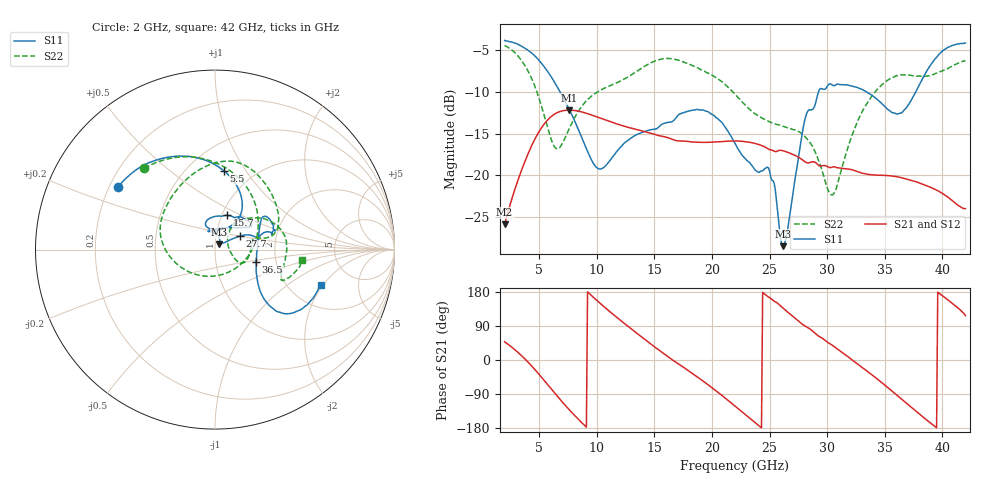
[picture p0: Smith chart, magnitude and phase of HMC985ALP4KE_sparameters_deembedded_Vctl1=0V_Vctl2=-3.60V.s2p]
!s2p File: Measurements: S11, S21, S12, S22
# GHz S dB R 50.0
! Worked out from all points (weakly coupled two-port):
!   401 points, 2 GHz to 42 GHz, reference 50 ohm
!   highest |S21| = -12.18 dB at 7.6 GHz (marker M1); lowest = -25.8 dB at 2 GHz (marker M2)
!   lowest |S11| = -28.5 dB at 26.2 GHz (marker M3), VSWR 1.08, Z = 52.3 + j3.11 ohm
!   |S11| at or under -10 dB: 6.815 GHz to 29.25 GHz (22.44 GHz wide, 124 % of centre); 33.42 GHz to 37.69 GHz (4.274 GHz wide, 12 % of centre)
!   |S22| runs from -22.3 to -4.4 dB; largest |S21 - S12| = 0.00033
!   S11 on the Smith chart (normalised r, x): 2 GHz: 0.24, +0.28; 5.5 GHz: 0.74, +0.80; 15.7 GHz: 1.06, +0.42; 27.7 GHz: 1.30, +0.20; 36.5 GHz: 1.57, -0.23; 42 GHz: 2.94, -1.90
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2  -3.84 146.9  -25.85 48.2  -25.85 48.1  -4.43 131.1
3.6  -4.63 120.0  -18.91 7.6  -18.91 7.6  -6.50 86.4
5.5  -7.10 83.4  -13.73 -56.3  -13.74 -56.3  -13.14 6.6
6.5  -9.23 66.2  -12.52 -92.8  -12.52 -92.8  -16.79 -67.9
7.6  -12.07 54.3  -12.18 -130.9  -12.19 -130.9  -14.43 -139.0
8.7  -15.47 54.6  -12.40 -165.5  -12.40 -165.5  -11.72 -173.2
10.3  -19.24 87.8  -13.13 149.3  -13.12 149.3  -9.80 160.8
12.6  -15.91 109.0  -14.20 91.5  -14.19 91.5  -8.29 127.3
15.4  -14.18 75.6  -15.25 26.3  -15.25 26.2  -6.14 85.0
15.7  -13.85 70.3  -15.31 19.6  -15.32 19.5  -6.04 81.3
19.4  -12.27 33.2  -16.04 -59.4  -16.04 -59.4  -7.57 35.0
22  -16.16 51.4  -15.87 -121.6  -15.88 -121.6  -10.28 12.9
24.9  -19.08 104.5  -16.85 166.4  -16.84 166.4  -13.51 12.0
26.2  -28.47 51.9  -17.05 136.2  -17.06 136.2  -14.13 -4.1
27.7  -16.15 28.7  -17.98 98.0  -17.98 97.9  -14.90 -22.9
28.7  -12.12 12.7  -18.37 77.3  -18.36 77.3  -16.45 -27.8
30.5  -9.22 18.3  -18.98 37.7  -18.99 37.7  -22.31 19.1
32.9  -9.63 33.9  -19.67 -16.7  -19.67 -16.7  -12.75 46.8
35.4  -12.22 11.7  -20.04 -76.1  -20.03 -76.1  -8.48 19.0
36.5  -12.48 -16.6  -20.29 -104.2  -20.29 -104.2  -7.96 6.0
39.5  -5.86 -43.7  -21.76 -178.6  -21.75 -178.7  -7.75 -24.2
42  -4.15 -18.6  -23.98 117.2  -23.98 117.1  -6.23 -6.9
